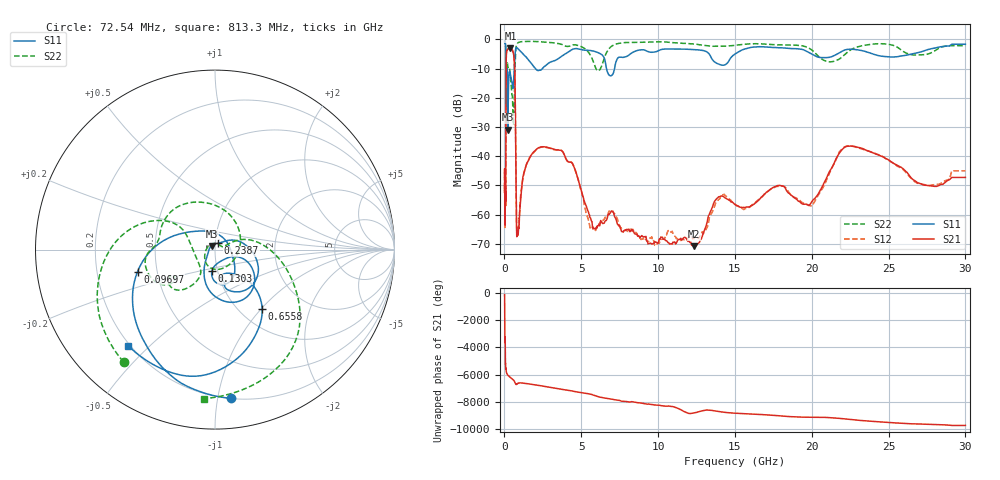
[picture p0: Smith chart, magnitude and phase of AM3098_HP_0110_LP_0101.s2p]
! Date/Time: Thu, Feb 28, 2019 8:37 AM
! Network Analyzer: Agilent Technologies E8364B Rev: A.07.50.67
! Sweep from 0.010 to 30.000 GHz, 1601 Points, Sweep Type: LOG
! Power Supply: 5.023 V, 0.002 A
# Hz S DB R 50
!freq MagS11 AngS11 MagS21 AngS21 MagS12 AngS12 MagS22 AngS22
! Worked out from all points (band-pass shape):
!   1601 points, 10 MHz to 30 GHz, reference 50 ohm
!   highest |S21| = -3.08 dB at 391.7 MHz (marker M1); lowest = -70.8 dB at 12.31 GHz (marker M2)
!   |S21| within 3 dB of the highest: 117.2 MHz to 618.8 MHz (501.5 MHz wide, 136 % of centre)
!   lowest |S11| = -30.9 dB at 230.5 MHz (marker M3), VSWR 1.06, Z = 48.1 + j2 ohm
!   |S11| at or under -10 dB: 175.9 MHz to 632.2 MHz (456.3 MHz wide, 113 % of centre); 2.023 GHz to 2.456 GHz (433.4 MHz wide, 19.4 % of centre); 6.641 GHz to 7.165 GHz (523.6 MHz wide, 7.58 % of centre)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
!   |S22| runs from -29.2 to -0.5 dB; largest |S21 - S12| = 0.0086
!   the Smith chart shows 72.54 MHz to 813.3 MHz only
!   S11 on the Smith chart (normalised r, x): 72.54 MHz: 0.20, -1.09; 96.97 MHz: 0.39, -0.12; 130.3 MHz: 0.94, -0.23; 238.7 MHz: 1.03, +0.07; 655.8 MHz: 1.26, -1.02; 813.3 MHz: 0.19, -0.43
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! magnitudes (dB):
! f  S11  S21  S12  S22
! 10 MHz  -0.3  -45.8  -47.7  -0.5
! 38.04 MHz  -0.5  -59.8  -58.4  -0.8
! 72.54 MHz  -1.6  -52.3  -54.5  -1.9
! 83.04 MHz  -2.5  -51.9  -50.0  -2.7
! 96.97 MHz  -7.0  -24.7  -24.6  -8.0
! 130.3 MHz  -18.3  -4.7  -4.7  -10.4
! 144.7 MHz  -18.4  -4.0  -3.9  -11.1
! 184.9 MHz  -10.8  -3.7  -3.6  -8.0
! 230.5 MHz  -30.9  -3.2  -3.2  -9.6
! 238.7 MHz  -28.0  -3.2  -3.1  -9.7
! 391.7 MHz  -12.1  -3.1  -3.1  -12.5
! 550.5 MHz  -16.8  -4.1  -4.1  -24.8
! 655.8 MHz  -7.5  -9.1  -9.1  -16.5
! 813.3 MHz  -2.8  -66.9  -65.1  -1.6
! 2.084 GHz  -10.4  -37.6  -37.6  -0.7
! 3.742 GHz  -5.6  -38.2  -38.2  -1.7
! 5.697 GHz  -3.9  -62.4  -64.3  -6.5
! 7.926 GHz  -5.9  -65.1  -65.4  -1.0
! 12.31 GHz  -3.5  -70.8  -68.1  -1.5
! 19.9 GHz  -4.7  -56.4  -56.9  -3.2
! 22.56 GHz  -3.3  -36.5  -36.5  -3.5
! 30 GHz  -1.7  -47.3  -45.0  -2.1
